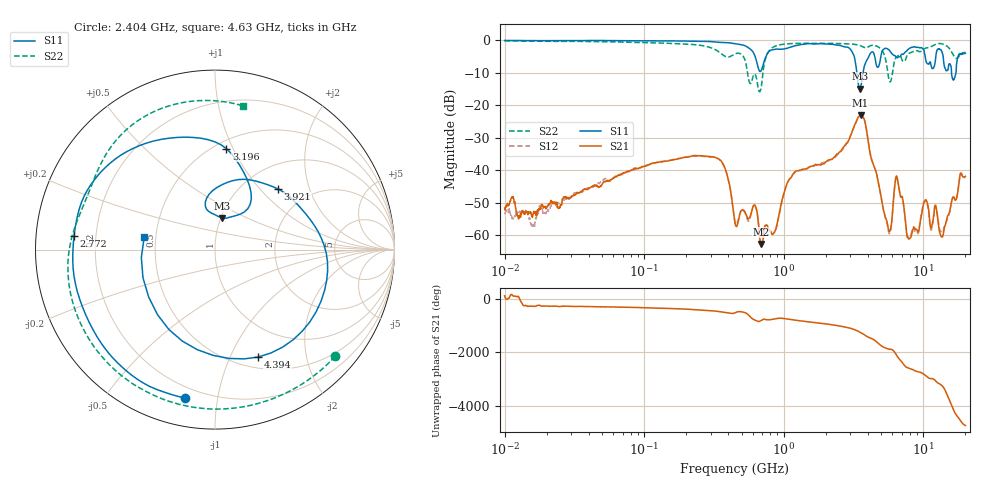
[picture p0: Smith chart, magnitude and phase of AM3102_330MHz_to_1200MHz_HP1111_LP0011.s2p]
! Date/Time: Tue, Sep 11, 2018 5:24 PM
! Network Analyzer: Agilent Technologies E8362B Rev: A.07.50.63
! Sweep from 0.010 to 20.000 GHz, 1601 Points, Sweep Type: LOG
! Power Supply: 4.949 V, 0.001 A
# Hz S DB R 50
!freq MagS11 AngS11 MagS21 AngS21 MagS12 AngS12 MagS22 AngS22
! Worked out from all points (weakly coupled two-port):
!   1601 points, 10 MHz to 20 GHz, reference 50 ohm
!   highest |S21| = -23.08 dB at 3.549 GHz (marker M1); lowest = -62.8 dB at 692.3 MHz (marker M2)
!   lowest |S11| = -14.9 dB at 3.498 GHz (marker M3), VSWR 1.44, Z = 50.8 + j18.3 ohm
!   |S11| at or under -10 dB: 3.338 GHz to 3.693 GHz (354.5 MHz wide, 10.1 % of centre); 15.91 GHz to 17.11 GHz (1.203 GHz wide, 7.28 % of centre)
!   |S22| runs from -15.8 to -0.1 dB; largest |S21 - S12| = 0.0056
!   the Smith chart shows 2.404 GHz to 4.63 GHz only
!   S11 on the Smith chart (normalised r, x): 2.404 GHz: 0.14, -0.81; 2.772 GHz: 0.12, +0.05; 3.196 GHz: 0.57, +0.94; 3.921 GHz: 1.43, +1.26; 4.394 GHz: 0.62, -1.28; 4.63 GHz: 0.43, +0.07
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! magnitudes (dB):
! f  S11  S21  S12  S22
! 10 MHz  0.0  -51.7  -53.3  -0.1
! 35.55 MHz  -0.1  -46.6  -46.8  -0.3
! 126.4 MHz  -0.2  -37.6  -37.6  -0.8
! 346 MHz  -0.6  -36.8  -36.8  -3.7
! 447.2 MHz  -1.0  -56.4  -55.9  -4.2
! 620.7 MHz  -4.8  -50.8  -50.9  -10.4
! 692.3 MHz  -9.1  -62.8  -63.4  -13.9
! 1.59 GHz  -1.1  -38.8  -38.8  -0.9
! 2.404 GHz  -1.5  -35.0  -35.5  -1.0
! 2.772 GHz  -2.1  -32.1  -32.4  -1.0
! 3.196 GHz  -4.9  -26.3  -26.4  -1.2
! 3.498 GHz  -14.9  -23.4  -23.2  -1.6
! 3.549 GHz  -14.4  -23.1  -23.0  -1.7
! 3.921 GHz  -6.2  -27.8  -27.8  -2.2
! 4.394 GHz  -3.8  -38.5  -38.4  -1.5
! 4.63 GHz  -7.9  -41.3  -41.4  -1.8
! 5.652 GHz  -2.9  -58.9  -59.3  -11.9
! 6.457 GHz  -5.3  -42.0  -42.2  -5.0
! 7.845 GHz  -2.7  -61.2  -60.6  -4.1
! 10.38 GHz  -5.9  -49.1  -49.3  -2.4
! 13.55 GHz  -3.4  -60.6  -59.1  -1.1
! 20 GHz  -4.0  -41.9  -42.5  -3.7
